| IBIS file stm32h562_563_573_vfqfpn68.ibs
[IBIS ver] 4.2
[File name] stm32h562_563_573_vfqfpn68.ibs
[File Rev] 1.1
[Date] 07-05-2024
[Source] Data Created at STMicroelectronics
[Notes]  File originated from ELDO simulations.
[Disclaimer]  This information is for modeling purpose only and is
   not guaranteed. The information is subject to change without
   notice.
[Copyright] Copyright 2024 STMicroelectronics Inc.
|   Component stm32h562_563_573_vfqfpn68
[Component] stm32h562_563_573_vfqfpn68
[Manufacturer] STMicroelectronics
[Package]
| variable   typ   min   max
R_pkg  0  NA  NA
L_pkg  0  NA  NA
C_pkg  0  NA  NA
[Pin]   signal_name   model_name
1  VBAT  power
2  PC13  io8_ft_i3c_spi
3  PC14-OSC32_IN  io8_ft_i3c_spi
4  PC15-OSC32_OUT  io8_ft_i3c_spi
5  PH0-OSC_IN  io8_ft_i3c_spi
6  PH1-OSC_OUT  io8_ft_i3c_spi
7  NRST  ioreset_ft_v33
8  PC0  io8_ft_spi
9  PC1  io8_ft_spi
10  PC2  io8_ft_spi
11  PC3  io8_ft_spi
12  VSSA  nc
13  VDDA  nc
14  PA0  io8_ft_spi
15  PA1  io8_ft_spi_tamp
16  PA2  io8_ft_spi
17  PA3  io8_ft_spi
18  VSS  gnd
19  VDD  power
20  PA4  io8_ft_spi
21  PA5  io8_ft_spi
22  PA6  io8_ft_spi
23  PA7  io8_ft_spi
24  PC4  io8_ft_spi
25  PC5  io8_ft_spi
26  PB0  io8_ft_spi
27  PB1  io8_ft_spi
28  PB2  io8_ft_i3c_spi
29  PB10  io8_ft_i3c_spi
30  PB11  io8_ft_i3c_spi
31  VCAP  nc
32  VSS  gnd
33  VDD  power
34  PB12  io8_ft_i3c_spi
|35  PB13  io8usb_ft_pd
|36  PB14  io8usb_ft_pd
35  PB13  nc
36  PB14  nc
37  PB15  io8_ft_spi
38  PD11  io8_ft_i3c_spi
39  PD12  io8_ft_i3c_spi
40  PC6  io8_ft_i3c_spi
41  PC7  io8_ft_i3c_spi
42  PC8  io8_ft_i3c_spi
43  PC9  io8_ft_i3c_spi
44  PA8  io8_ft_i3c_spi
45  PA9  io8_ft_i3c_spi
46  PA10  io8_ft_i3c_spi
47  PA11  io8usb_ft_i3c_spi_phy
48  PA12  io8usb_ft_i3c_spi_phy
49  PA13  io8_ft_i3c_spi
50  VSS  gnd
51  VDD  power
52  PA14  io8_ft_i3c_spi
53  PA15  io8_ft_i3c_spi
54  PC10  io8_ft_i3c_spi
55  PC11  io8_ft_i3c_spi
56  PC12  io8_ft_i3c_spi
57  PB3  io8_ft_i3c_spi
58  PB4  io8_ft_i3c_spi
59  PB5  io8_ft_i3c_spi
60  PB6  io8_ft_i3c_spi
61  PB7  io8_ft_i3c_spi
62  BOOT0  vpphv
63  PB8  io8_ft_i3c_spi
64  PB9  io8_ft_i3c_spi
65  PE0  io8_ft_i3c_spi
66  VCAP  nc
67  VSS  gnd
68  VDD  power
0  VSS  gnd
[Package Model]   484-vfqfpn-8x8-68-ldo-221014
[Pin Mapping]   pulldown_ref   pullup_ref   | Comment
1  nc  vsw
2  gndio  vddiom  | Depending on IO usage
| 2  gndio  vsw  | Depending on IO usage
3  gndio  vddiom  | Depending on IO usage
| 3  gndio  vsw  | Depending on IO usage
4  gndio  vddiom  | Depending on IO usage
| 4  gndio  vsw  | Depending on IO usage
5  gndio  vddiom
6  gndio  vddiom
7  gndio  vddiom
8  gndio  vddiom
9  gndio  vddiom
10  gndio  vddiom
11  gndio  vddiom
12  nc  nc
13  nc  nc
14  gndio  vddiom
15  gndio  vddiom
16  gndio  vddiom
17  gndio  vddiom
18  gndio  nc
19  nc  vddiom
20  gndio  vddiom
21  gndio  vddiom
22  gndio  vddiom
23  gndio  vddiom
24  gndio  vddiom
25  gndio  vddiom
26  gndio  vddiom
27  gndio  vddiom
28  gndio  vddiom
29  gndio  vddiom
30  gndio  vddiom
31  nc  nc
32  gndio  nc
33  nc  vddiom
34  gndio  vddiom
|35  gndio  vddiom
35  nc nc
|36  gndio  vddiom
36  nc nc
37  gndio  vddiom
38  gndio  vddiom
39  gndio  vddiom
40  gndio  vddiom
41  gndio  vddiom
42  gndio  vddiom
43  gndio  vddiom
44  gndio  vddiom
45  gndio  vddiom
46  gndio  vddiom
47  gndio  vddiom
48  gndio  vddiom
49  gndio  vddiom
50  gndio  nc
51  nc  vddiom
52  gndio  vddiom
53  gndio  vddiom
54  gndio  vddiom
55  gndio  vddiom
56  gndio  vddiom
57  gndio  vddiom
58  gndio  vddiom
59  gndio  vddiom
60  gndio  vddiom
61  gndio  vddiom
62  gndio  vddiom
63  gndio  vddiom
64  gndio  vddiom
65  gndio  vddiom
66  nc  nc
67  gndio  nc
68  nc  vddiom
0  gndio  nc
[Model Selector] io8_ft_i3c_spi
io8_ft_spi_ls_1v2 "io8_ft spi low speed @ 1.2V"
io8_ft_spi_ls_1v8 "io8_ft spi low speed @ 1.8V"
io8_ft_spi_ls_3v3 "io8_ft spi low speed @ 3.3V"
io8_ft_spi_ms_1v2 "io8_ft spi med speed @ 1.2V"
io8_ft_spi_ms_1v8 "io8_ft spi med speed @ 1.8V"
io8_ft_spi_ms_3v3 "io8_ft spi med speed @ 3.3V"
io8_ft_spi_fs_1v2 "io8_ft spi fast speed @ 1.2V"
io8_ft_spi_fs_1v8 "io8_ft spi fast speed @ 1.8V"
io8_ft_spi_fs_3v3 "io8_ft spi fast speed @ 3.3V"
io8_ft_spi_hs_1v2 "io8_ft spi high speed @ 1.2V"
io8_ft_spi_hs_1v8 "io8_ft spi high speed @ 1.8V"
io8_ft_spi_hs_3v3 "io8_ft spi high speed @ 3.3V"
io8_ft_hslv_spi_ls_1v2 "io8_ft spi hslv low speed @ 1.2V"
io8_ft_hslv_spi_ls_1v8 "io8_ft spi hslv low speed @ 1.8V"
io8_ft_hslv_spi_ls_2v5 "io8_ft spi hslv low speed @ 2.5V"
io8_ft_hslv_spi_ms_1v2 "io8_ft spi hslv med speed @ 1.2V"
io8_ft_hslv_spi_ms_1v8 "io8_ft spi hslv med speed @ 1.8V"
io8_ft_hslv_spi_ms_2v5 "io8_ft spi hslv med speed @ 2.5V"
io8_ft_hslv_spi_fs_1v2 "io8_ft spi hslv fast speed @ 1.2V"
io8_ft_hslv_spi_fs_1v8 "io8_ft spi hslv fast speed @ 1.8V"
io8_ft_hslv_spi_fs_2v5 "io8_ft spi hslv fast speed @ 2.5V"
io8_ft_hslv_spi_hs_1v2 "io8_ft spi hslv high speed @ 1.2V"
io8_ft_hslv_spi_hs_1v8 "io8_ft spi hslv high speed @ 1.8V"
io8_ft_hslv_spi_hs_2v5 "io8_ft spi hslv high speed @ 2.5V"
io8_ft_i3c_spi_ls_1v2 "io8_ft i3c spi open-drain low speed @ 1.2V"
io8_ft_i3c_spi_ls_1v8 "io8_ft i3c spi open-drain low speed @ 1.8V"
io8_ft_i3c_spi_ls_3v3 "io8_ft i3c spi open-drain low speed @ 3.3V"
io8_ft_i3c_spi_ms_1v2 "io8_ft i3c spi open-drain med speed @ 1.2V"
io8_ft_i3c_spi_ms_1v8 "io8_ft i3c spi open-drain med speed @ 1.8V"
io8_ft_i3c_spi_ms_3v3 "io8_ft i3c spi open-drain med speed @ 3.3V"
io8_ft_i3c_spi_fs_1v2 "io8_ft i3c spi open-drain fast speed @ 1.2V"
io8_ft_i3c_spi_fs_1v8 "io8_ft i3c spi open-drain fast speed @ 1.8V"
io8_ft_i3c_spi_fs_3v3 "io8_ft i3c spi open-drain fast speed @ 3.3V"
io8_ft_i3c_spi_hs_1v2 "io8_ft i3c spi open-drain high speed @ 1.2V"
io8_ft_i3c_spi_hs_1v8 "io8_ft i3c spi open-drain high speed @ 1.8V"
io8_ft_i3c_spi_hs_3v3 "io8_ft i3c spi open-drain high speed @ 3.3V"
io8_ft_hslv_i3c_spi_ls_1v2 "io8_ft hslv i3c spi open-drain low speed @ 1.2V"
io8_ft_hslv_i3c_spi_ls_1v8 "io8_ft hslv i3c spi open-drain low speed @ 1.8V"
io8_ft_hslv_i3c_spi_ls_2v5 "io8_ft hslv i3c spi open-drain low speed @ 2.5V"
io8_ft_hslv_i3c_spi_ms_1v2 "io8_ft hslv i3c spi open-drain med speed @ 1.2V"
io8_ft_hslv_i3c_spi_ms_1v8 "io8_ft hslv i3c spi open-drain med speed @ 1.8V"
io8_ft_hslv_i3c_spi_ms_2v5 "io8_ft hslv i3c spi open-drain med speed @ 2.5V"
io8_ft_hslv_i3c_spi_fs_1v2 "io8_ft hslv i3c spi open-drain fast speed @ 1.2V"
io8_ft_hslv_i3c_spi_fs_1v8 "io8_ft hslv i3c spi open-drain fast speed @ 1.8V"
io8_ft_hslv_i3c_spi_fs_2v5 "io8_ft hslv i3c spi open-drain fast speed @ 2.5V"
io8_ft_hslv_i3c_spi_hs_1v2 "io8_ft hslv i3c spi open-drain high speed @ 1.2V"
io8_ft_hslv_i3c_spi_hs_1v8 "io8_ft hslv i3c spi open-drain high speed @ 1.8V"
io8_ft_hslv_i3c_spi_hs_2v5 "io8_ft hslv i3c spi open-drain high speed @ 2.5V"
io8_ft_i3c_fmp_spi_3v3 "io8_ft i3c fm+ spi open-drain @ 3.3V"
io8_ft_i3c_fmp_spi_1v8 "io8_ft i3c fm+ spi open-drain @ 1.8V"
io8_ft_i3c_fmp_spi_1v2 "io8_ft i3c fm+ spi open-drain @ 1.2V"
[Model Selector] io8_ft_spi
io8_ft_spi_ls_1v2 "io8_ft spi low speed @ 1.2V"
io8_ft_spi_ls_1v8 "io8_ft spi low speed @ 1.8V"
io8_ft_spi_ls_3v3 "io8_ft spi low speed @ 3.3V"
io8_ft_spi_ms_1v2 "io8_ft spi med speed @ 1.2V"
io8_ft_spi_ms_1v8 "io8_ft spi med speed @ 1.8V"
io8_ft_spi_ms_3v3 "io8_ft spi med speed @ 3.3V"
io8_ft_spi_fs_1v2 "io8_ft spi fast speed @ 1.2V"
io8_ft_spi_fs_1v8 "io8_ft spi fast speed @ 1.8V"
io8_ft_spi_fs_3v3 "io8_ft spi fast speed @ 3.3V"
io8_ft_spi_hs_1v2 "io8_ft spi high speed @ 1.2V"
io8_ft_spi_hs_1v8 "io8_ft spi high speed @ 1.8V"
io8_ft_spi_hs_3v3 "io8_ft spi high speed @ 3.3V"
io8_ft_hslv_spi_ls_1v2 "io8_ft spi hslv low speed @ 1.2V"
io8_ft_hslv_spi_ls_1v8 "io8_ft spi hslv low speed @ 1.8V"
io8_ft_hslv_spi_ls_2v5 "io8_ft spi hslv low speed @ 2.5V"
io8_ft_hslv_spi_ms_1v2 "io8_ft spi hslv med speed @ 1.2V"
io8_ft_hslv_spi_ms_1v8 "io8_ft spi hslv med speed @ 1.8V"
io8_ft_hslv_spi_ms_2v5 "io8_ft spi hslv med speed @ 2.5V"
io8_ft_hslv_spi_fs_1v2 "io8_ft spi hslv fast speed @ 1.2V"
io8_ft_hslv_spi_fs_1v8 "io8_ft spi hslv fast speed @ 1.8V"
io8_ft_hslv_spi_fs_2v5 "io8_ft spi hslv fast speed @ 2.5V"
io8_ft_hslv_spi_hs_1v2 "io8_ft spi hslv high speed @ 1.2V"
io8_ft_hslv_spi_hs_1v8 "io8_ft spi hslv high speed @ 1.8V"
io8_ft_hslv_spi_hs_2v5 "io8_ft spi hslv high speed @ 2.5V"
[Model Selector] io8_ft_spi_tamp
io8_ft_spi_ls_1v2 "io8_ft spi low speed @ 1.2V"
io8_ft_spi_ls_1v8 "io8_ft spi low speed @ 1.8V"
io8_ft_spi_ls_3v3 "io8_ft spi low speed @ 3.3V"
io8_ft_spi_ms_1v2 "io8_ft spi med speed @ 1.2V"
io8_ft_spi_ms_1v8 "io8_ft spi med speed @ 1.8V"
io8_ft_spi_ms_3v3 "io8_ft spi med speed @ 3.3V"
io8_ft_spi_fs_1v2 "io8_ft spi fast speed @ 1.2V"
io8_ft_spi_fs_1v8 "io8_ft spi fast speed @ 1.8V"
io8_ft_spi_fs_3v3 "io8_ft spi fast speed @ 3.3V"
io8_ft_spi_hs_1v2 "io8_ft spi high speed @ 1.2V"
io8_ft_spi_hs_1v8 "io8_ft spi high speed @ 1.8V"
io8_ft_spi_hs_3v3 "io8_ft spi high speed @ 3.3V"
io8_ft_hslv_spi_ls_1v2 "io8_ft spi hslv low speed @ 1.2V"
io8_ft_hslv_spi_ls_1v8 "io8_ft spi hslv low speed @ 1.8V"
io8_ft_hslv_spi_ls_2v5 "io8_ft spi hslv low speed @ 2.5V"
io8_ft_hslv_spi_ms_1v2 "io8_ft spi hslv med speed @ 1.2V"
io8_ft_hslv_spi_ms_1v8 "io8_ft spi hslv med speed @ 1.8V"
io8_ft_hslv_spi_ms_2v5 "io8_ft spi hslv med speed @ 2.5V"
io8_ft_hslv_spi_fs_1v2 "io8_ft spi hslv fast speed @ 1.2V"
io8_ft_hslv_spi_fs_1v8 "io8_ft spi hslv fast speed @ 1.8V"
io8_ft_hslv_spi_fs_2v5 "io8_ft spi hslv fast speed @ 2.5V"
io8_ft_hslv_spi_hs_1v2 "io8_ft spi hslv high speed @ 1.2V"
io8_ft_hslv_spi_hs_1v8 "io8_ft spi hslv high speed @ 1.8V"
io8_ft_hslv_spi_hs_2v5 "io8_ft spi hslv high speed @ 2.5V"
io8_ft_tamp_v33_1v2 "io8_ft tamp V33 @ 1.2V"
io8_ft_tamp_v33_1v8 "io8_ft tamp V33 @ 1.2V"
io8_ft_tamp_v33_3v3 "io8_ft tamp V33 @ 1.2V"
[Model Selector] io8usb_ft_i3c_spi_phy
io8_ft_spi_ls_1v2 "io8_ft spi low speed @ 1.2V"
io8_ft_spi_ls_1v8 "io8_ft spi low speed @ 1.8V"
io8_ft_spi_ls_3v3 "io8_ft spi low speed @ 3.3V"
io8_ft_spi_ms_1v2 "io8_ft spi med speed @ 1.2V"
io8_ft_spi_ms_1v8 "io8_ft spi med speed @ 1.8V"
io8_ft_spi_ms_3v3 "io8_ft spi med speed @ 3.3V"
io8_ft_spi_fs_1v2 "io8_ft spi fast speed @ 1.2V"
io8_ft_spi_fs_1v8 "io8_ft spi fast speed @ 1.8V"
io8_ft_spi_fs_3v3 "io8_ft spi fast speed @ 3.3V"
io8_ft_spi_hs_1v2 "io8_ft spi high speed @ 1.2V"
io8_ft_spi_hs_1v8 "io8_ft spi high speed @ 1.8V"
io8_ft_spi_hs_3v3 "io8_ft spi high speed @ 3.3V"
io8_ft_hslv_spi_ls_1v2 "io8_ft spi hslv low speed @ 1.2V"
io8_ft_hslv_spi_ls_1v8 "io8_ft spi hslv low speed @ 1.8V"
io8_ft_hslv_spi_ls_2v5 "io8_ft spi hslv low speed @ 2.5V"
io8_ft_hslv_spi_ms_1v2 "io8_ft spi hslv med speed @ 1.2V"
io8_ft_hslv_spi_ms_1v8 "io8_ft spi hslv med speed @ 1.8V"
io8_ft_hslv_spi_ms_2v5 "io8_ft spi hslv med speed @ 2.5V"
io8_ft_hslv_spi_fs_1v2 "io8_ft spi hslv fast speed @ 1.2V"
io8_ft_hslv_spi_fs_1v8 "io8_ft spi hslv fast speed @ 1.8V"
io8_ft_hslv_spi_fs_2v5 "io8_ft spi hslv fast speed @ 2.5V"
io8_ft_hslv_spi_hs_1v2 "io8_ft spi hslv high speed @ 1.2V"
io8_ft_hslv_spi_hs_1v8 "io8_ft spi hslv high speed @ 1.8V"
io8_ft_hslv_spi_hs_2v5 "io8_ft spi hslv high speed @ 2.5V"
io8_ft_i3c_spi_ls_1v2 "io8_ft i3c spi open-drain low speed @ 1.2V"
io8_ft_i3c_spi_ls_1v8 "io8_ft i3c spi open-drain low speed @ 1.8V"
io8_ft_i3c_spi_ls_3v3 "io8_ft i3c spi open-drain low speed @ 3.3V"
io8_ft_i3c_spi_ms_1v2 "io8_ft i3c spi open-drain med speed @ 1.2V"
io8_ft_i3c_spi_ms_1v8 "io8_ft i3c spi open-drain med speed @ 1.8V"
io8_ft_i3c_spi_ms_3v3 "io8_ft i3c spi open-drain med speed @ 3.3V"
io8_ft_i3c_spi_fs_1v2 "io8_ft i3c spi open-drain fast speed @ 1.2V"
io8_ft_i3c_spi_fs_1v8 "io8_ft i3c spi open-drain fast speed @ 1.8V"
io8_ft_i3c_spi_fs_3v3 "io8_ft i3c spi open-drain fast speed @ 3.3V"
io8_ft_i3c_spi_hs_1v2 "io8_ft i3c spi open-drain high speed @ 1.2V"
io8_ft_i3c_spi_hs_1v8 "io8_ft i3c spi open-drain high speed @ 1.8V"
io8_ft_i3c_spi_hs_3v3 "io8_ft i3c spi open-drain high speed @ 3.3V"
io8_ft_hslv_i3c_spi_ls_1v2 "io8_ft hslv i3c spi open-drain low speed @ 1.2V"
io8_ft_hslv_i3c_spi_ls_1v8 "io8_ft hslv i3c spi open-drain low speed @ 1.8V"
io8_ft_hslv_i3c_spi_ls_2v5 "io8_ft hslv i3c spi open-drain low speed @ 2.5V"
io8_ft_hslv_i3c_spi_ms_1v2 "io8_ft hslv i3c spi open-drain med speed @ 1.2V"
io8_ft_hslv_i3c_spi_ms_1v8 "io8_ft hslv i3c spi open-drain med speed @ 1.8V"
io8_ft_hslv_i3c_spi_ms_2v5 "io8_ft hslv i3c spi open-drain med speed @ 2.5V"
io8_ft_hslv_i3c_spi_fs_1v2 "io8_ft hslv i3c spi open-drain fast speed @ 1.2V"
io8_ft_hslv_i3c_spi_fs_1v8 "io8_ft hslv i3c spi open-drain fast speed @ 1.8V"
io8_ft_hslv_i3c_spi_fs_2v5 "io8_ft hslv i3c spi open-drain fast speed @ 2.5V"
io8_ft_hslv_i3c_spi_hs_1v2 "io8_ft hslv i3c spi open-drain high speed @ 1.2V"
io8_ft_hslv_i3c_spi_hs_1v8 "io8_ft hslv i3c spi open-drain high speed @ 1.8V"
io8_ft_hslv_i3c_spi_hs_2v5 "io8_ft hslv i3c spi open-drain high speed @ 2.5V"
io8_ft_i3c_fmp_spi_3v3 "io8_ft i3c fm+ spi open-drain @ 3.3V"
io8_ft_i3c_fmp_spi_1v8 "io8_ft i3c fm+ spi open-drain @ 1.8V"
io8_ft_i3c_fmp_spi_1v2 "io8_ft i3c fm+ spi open-drain @ 1.2V"
io8usb_ft_phy_ls_2v5 "iousb ft low speed @ 2.5V"
io8usb_ft_phy_ls_3v3 "iousb ft low speed @ 3.3V"
io8usb_ft_phy_fs_2v5 "iousb ft fast speed @ 2.5V"
io8usb_ft_phy_fs_3v3 "iousb ft fast speed @ 3.3V"
[Model Selector] ioreset_ft_v33
ioreset_ft_v33_1v2 "Reset PAD. 5V tolerant. 1.2V range"
ioreset_ft_v33_1v8 "Reset PAD. 5V tolerant. 1.8V range"
ioreset_ft_v33_3v3 "Reset PAD. 5V tolerant. 3.3V range"
[Model Selector] vpphv
vpphv_1v2 "Flash Test cell v33 = 1.2 V range"
vpphv_1v8 "Flash Test cell v33 = 1.8 V range"
vpphv_3v3 "Flash Test cell v33 = 3.3 V range"
[Define Package Model]  484-vfqfpn-8x8-68-ldo-221014
[Manufacturer]  Unknown
[OEM]  Unknown
[Description]  None
[Number Of Pins]  65
[Pin Numbers]
| Pin Num   Terminal Name
7 | NRST
14 | PA0
15 | PA1
16 | PA2
17 | PA3
20 | PA4
21 | PA5
22 | PA6
23 | PA7
44 | PA8
45 | PA9
46 | PA10
47 | PA11
48 | PA12
49 | PA13
52 | PA14
53 | PA15
26 | PB0
27 | PB1
28 | PB2
57 | PB3
58 | PB4
59 | PB5
60 | PB6
61 | PB7
63 | PB8
64 | PB9
29 | PB10
30 | PB11
34 | PB12
35 | PB13
36 | PB14
37 | PB15
8 | PC0
9 | PC1
10 | PC2
11 | PC3
24 | PC4
25 | PC5
40 | PC6
41 | PC7
42 | PC8
43 | PC9
54 | PC10
55 | PC11
56 | PC12
2 | PC13
3 | PC14-OSC32_IN
4 | PC15-OSC32_OUT
38 | PD11
39 | PD12
65 | PE0
5 | PH0-OSC_IN
6 | PH1-OSC_OUT
1 | VBAT
31 | VCAP
66 | VCAP
33 | VDD
51 | VDD
19 | VDD
68 | VDD
13 | VDDA
62 | BOOT0
18 | VSS
12 | VSSA
|[Merged Pins]  18
|32  |  VSS
|50  |  VSS
|67  |  VSS
[Model Data]
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[End Model Data]
[End Package Model]
|End [Component]
| Models and submodels in the file (64): io8_ft_hslv_i3c_spi_fs_1v2 (I/O_open_drain), io8_ft_hslv_i3c_spi_fs_1v8 (I/O_open_drain), io8_ft_hslv_i3c_spi_fs_2v5 (I/O_open_drain), io8_ft_hslv_i3c_spi_hs_1v2 (I/O_open_drain), io8_ft_hslv_i3c_spi_hs_1v8 (I/O_open_drain), io8_ft_hslv_i3c_spi_hs_2v5 (I/O_open_drain), io8_ft_hslv_i3c_spi_ls_1v2 (I/O_open_drain), io8_ft_hslv_i3c_spi_ls_1v8 (I/O_open_drain), io8_ft_hslv_i3c_spi_ls_2v5 (I/O_open_drain), io8_ft_hslv_i3c_spi_ms_1v2 (I/O_open_drain), io8_ft_hslv_i3c_spi_ms_1v8 (I/O_open_drain), io8_ft_hslv_i3c_spi_ms_2v5 (I/O_open_drain), io8_ft_hslv_spi_fs_1v2 (I/O), io8_ft_hslv_spi_fs_1v8 (I/O), io8_ft_hslv_spi_fs_2v5 (I/O), io8_ft_hslv_spi_hs_1v2 (I/O), io8_ft_hslv_spi_hs_1v8 (I/O), io8_ft_hslv_spi_hs_2v5 (I/O), io8_ft_hslv_spi_ls_1v2 (I/O), io8_ft_hslv_spi_ls_1v8 (I/O), io8_ft_hslv_spi_ls_2v5 (I/O), io8_ft_hslv_spi_ms_1v2 (I/O), io8_ft_hslv_spi_ms_1v8 (I/O), io8_ft_hslv_spi_ms_2v5 (I/O), io8_ft_i3c_fmp_spi_1v2 (I/O_open_drain), io8_ft_i3c_fmp_spi_1v8 (I/O_open_drain), io8_ft_i3c_fmp_spi_3v3 (I/O_open_drain), io8_ft_i3c_spi_fs_1v2 (I/O_open_drain), io8_ft_i3c_spi_fs_1v8 (I/O_open_drain), io8_ft_i3c_spi_fs_3v3 (I/O_open_drain), io8_ft_i3c_spi_hs_1v2 (I/O_open_drain), io8_ft_i3c_spi_hs_1v8 (I/O_open_drain), io8_ft_i3c_spi_hs_3v3 (I/O_open_drain), io8_ft_i3c_spi_ls_1v2 (I/O_open_drain), io8_ft_i3c_spi_ls_1v8 (I/O_open_drain), io8_ft_i3c_spi_ls_3v3 (I/O_open_drain), io8_ft_i3c_spi_ms_1v2 (I/O_open_drain), io8_ft_i3c_spi_ms_1v8 (I/O_open_drain), io8_ft_i3c_spi_ms_3v3 (I/O_open_drain), io8_ft_spi_fs_1v2 (I/O), io8_ft_spi_fs_1v8 (I/O), io8_ft_spi_fs_3v3 (I/O), io8_ft_spi_hs_1v2 (I/O), io8_ft_spi_hs_1v8 (I/O), io8_ft_spi_hs_3v3 (I/O), io8_ft_spi_ls_1v2 (I/O), io8_ft_spi_ls_1v8 (I/O), io8_ft_spi_ls_3v3 (I/O), io8_ft_spi_ms_1v2 (I/O), io8_ft_spi_ms_1v8 (I/O), io8_ft_spi_ms_3v3 (I/O), io8_ft_tamp_v33_1v2 (I/O), io8_ft_tamp_v33_1v8 (I/O), io8_ft_tamp_v33_3v3 (I/O), io8usb_ft_phy_fs_2v5 (I/O), io8usb_ft_phy_fs_3v3 (I/O), io8usb_ft_phy_ls_2v5 (I/O), io8usb_ft_phy_ls_3v3 (I/O), ioreset_ft_v33_1v2 (I/O_open_drain), ioreset_ft_v33_1v8 (I/O_open_drain), ioreset_ft_v33_3v3 (I/O_open_drain), vpphv_1v2 (Input), vpphv_1v8 (Input), vpphv_3v3 (Input)
